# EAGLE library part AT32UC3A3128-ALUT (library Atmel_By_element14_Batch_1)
32-bit Microcontroller
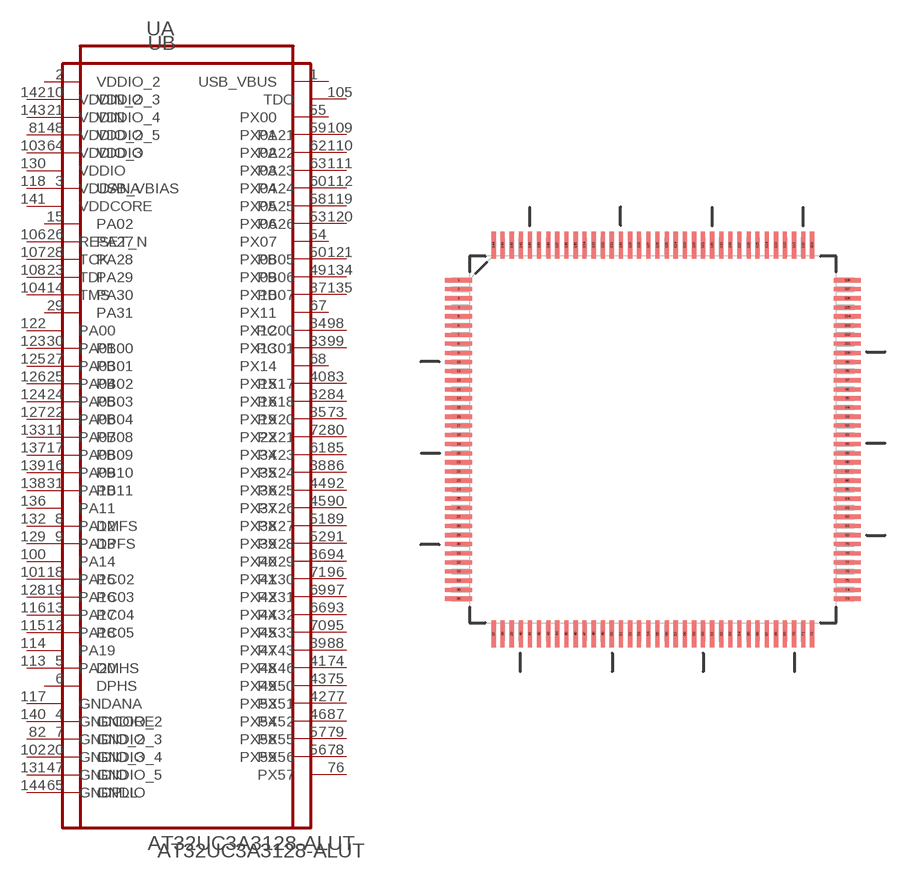
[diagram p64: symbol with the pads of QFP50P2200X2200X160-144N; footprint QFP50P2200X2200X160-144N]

Designator prefix U; gates A=AT32UC3A3128-ALUT_A B=AT32UC3A3128-ALUT_B

## AT32UC3A3128-ALUT (DESCRIPTION: 32-bit Microcontroller; MPN: AT32UC3A3128-ALUT; OC_FARNELL: 1841638; OC_NEWARK: 12T1371; PACKAGE: LQFP-144; SUPPLIER: Atmel Corporation)  [QFP50P2200X2200X160-144N]
1  A:USB_VBUS  out
2  A:VDDIO_2  pwr
3  A:USB_VBIAS  pas
4  A:GNDIO_2  pas
5  A:DMHS  pas
6  A:DPHS  pas
7  A:GNDIO_3  pas
8  A:DMFS
9  A:DPFS
10  A:VDDIO_3  pwr
11  A:PB08
12  A:PC05
13  A:PC04
14  A:PA30
15  A:PA02
16  A:PB10
17  A:PB09
18  A:PC02
19  A:PC03
20  A:GNDIO_4  pas
21  A:VDDIO_4  pwr
22  A:PB04
23  A:PA29
24  A:PB03
25  A:PB02
26  A:PA27
27  A:PB01
28  A:PA28
29  A:PA31
30  A:PB00
31  A:PB11
32  A:PX16
33  A:PX13
34  A:PX12
35  A:PX19
36  A:PX40
37  A:PX10
38  A:PX35
39  A:PX47
40  A:PX15
41  A:PX48
42  A:PX53
43  A:PX49
44  A:PX36
45  A:PX37
46  A:PX54
47  A:GNDIO_5  pas
48  A:VDDIO_5  pwr
49  A:PX09
50  A:PX08
51  A:PX38
52  A:PX39
53  A:PX06
54  A:PX07
55  A:PX00
56  A:PX59
57  A:PX58
58  A:PX05
59  A:PX01
60  A:PX04
61  A:PX34
62  A:PX02
63  A:PX03
64  A:VDDIO  pwr
65  A:GNDIO  pas
66  A:PX44
67  A:PX11
68  A:PX14
69  A:PX42
70  A:PX45
71  A:PX41
72  A:PX22
73  B:PX20
74  B:PX46
75  B:PX50
76  B:PX57
77  B:PX51
78  B:PX56
79  B:PX55
80  B:PX21
81  B:VDDIO_2  pwr
82  B:GNDIO_2  pas
83  B:PX17
84  B:PX18
85  B:PX23
86  B:PX24
87  B:PX52
88  B:PX43
89  B:PX27
90  B:PX26
91  B:PX28
92  B:PX25
93  B:PX32
94  B:PX29
95  B:PX33
96  B:PX30
97  B:PX31
98  B:PC00
99  B:PC01
100  B:PA14
101  B:PA15
102  B:GNDIO_3  pas
103  B:VDDIO_3  pwr
104  B:TMS  in
105  B:TDO  out
106  B:RESET_N  in
107  B:TCK  in
108  B:TDI  in
109  B:PA21
110  B:PA22
111  B:PA23
112  B:PA24
113  B:PA20
114  B:PA19
115  B:PA18
116  B:PA17
117  B:GNDANA  pas
118  B:VDDANA  pwr
119  B:PA25
120  B:PA26
121  B:PB05
122  B:PA00
123  B:PA01
124  B:PA05
125  B:PA03
126  B:PA04
127  B:PA06
128  B:PA16
129  B:PA13
130  B:VDDIO  pwr
131  B:GNDIO  pas
132  B:PA12
133  B:PA07
134  B:PB06
135  B:PB07
136  B:PA11
137  B:PA08
138  B:PA10
139  B:PA09
140  B:GNDCORE  pas
141  B:VDDCORE  pwr
142  B:VDDIN_2  pwr
143  B:VDDIN  pwr
144  B:GNDPLL  pas

## Footprint QFP50P2200X2200X160-144N (pad centres in mm)
smd 1.473 x 0.229: 1 -10.668,8.738; 2 -10.668,8.255; 3 -10.668,7.747; 4 -10.668,7.239; 5 -10.668,6.756; 6 -10.668,6.248; 7 -10.668,5.74; 8 -10.668,5.258; 9 -10.668,4.75; 10 -10.668,4.242; 11 -10.668,3.759; 12 -10.668,3.251; 13 -10.668,2.743; 14 -10.668,2.261; 15 -10.668,1.753; 16 -10.668,1.245; 17 -10.668,0.762; 18 -10.668,0.254; 19 -10.668,-0.254; 20 -10.668,-0.762; 21 -10.668,-1.245; 22 -10.668,-1.753; 23 -10.668,-2.261; 24 -10.668,-2.743; 25 -10.668,-3.251; 26 -10.668,-3.759; 27 -10.668,-4.242; 28 -10.668,-4.75; 29 -10.668,-5.258; 30 -10.668,-5.74; 31 -10.668,-6.248; 32 -10.668,-6.756; 33 -10.668,-7.239; 34 -10.668,-7.747; 35 -10.668,-8.255; 36 -10.668,-8.738; 73 10.668,-8.738; 74 10.668,-8.255; 75 10.668,-7.747; 76 10.668,-7.239; 77 10.668,-6.756; 78 10.668,-6.248; 79 10.668,-5.74; 80 10.668,-5.258; 81 10.668,-4.75; 82 10.668,-4.242; 83 10.668,-3.759; 84 10.668,-3.251; 85 10.668,-2.743; 86 10.668,-2.261; 87 10.668,-1.753; 88 10.668,-1.245; 89 10.668,-0.762; 90 10.668,-0.254; 91 10.668,0.254; 92 10.668,0.762; 93 10.668,1.245; 94 10.668,1.753; 95 10.668,2.261; 96 10.668,2.743; 97 10.668,3.251; 98 10.668,3.759; 99 10.668,4.242; 100 10.668,4.75; 101 10.668,5.258; 102 10.668,5.74; 103 10.668,6.248; 104 10.668,6.756; 105 10.668,7.239; 106 10.668,7.747; 107 10.668,8.255; 108 10.668,8.738
smd 0.229 x 1.473: 37 -8.738,-10.668; 38 -8.255,-10.668; 39 -7.747,-10.668; 40 -7.239,-10.668; 41 -6.756,-10.668; 42 -6.248,-10.668; 43 -5.74,-10.668; 44 -5.258,-10.668; 45 -4.75,-10.668; 46 -4.242,-10.668; 47 -3.759,-10.668; 48 -3.251,-10.668; 49 -2.743,-10.668; 50 -2.261,-10.668; 51 -1.753,-10.668; 52 -1.245,-10.668; 53 -0.762,-10.668; 54 -0.254,-10.668; 55 0.254,-10.668; 56 0.762,-10.668; 57 1.245,-10.668; 58 1.753,-10.668; 59 2.261,-10.668; 60 2.743,-10.668; 61 3.251,-10.668; 62 3.759,-10.668; 63 4.242,-10.668; 64 4.75,-10.668; 65 5.258,-10.668; 66 5.74,-10.668; 67 6.248,-10.668; 68 6.756,-10.668; 69 7.239,-10.668; 70 7.747,-10.668; 71 8.255,-10.668; 72 8.738,-10.668; 109 8.738,10.668; 110 8.255,10.668; 111 7.747,10.668; 112 7.239,10.668; 113 6.756,10.668; 114 6.248,10.668; 115 5.74,10.668; 116 5.258,10.668; 117 4.75,10.668; 118 4.242,10.668; 119 3.759,10.668; 120 3.251,10.668; 121 2.743,10.668; 122 2.261,10.668; 123 1.753,10.668; 124 1.245,10.668; 125 0.762,10.668; 126 0.254,10.668; 127 -0.254,10.668; 128 -0.762,10.668; 129 -1.245,10.668; 130 -1.753,10.668; 131 -2.261,10.668; 132 -2.743,10.668; 133 -3.251,10.668; 134 -3.759,10.668; 135 -4.242,10.668; 136 -4.75,10.668; 137 -5.258,10.668; 138 -5.74,10.668; 139 -6.248,10.668; 140 -6.756,10.668; 141 -7.239,10.668; 142 -7.747,10.668; 143 -8.255,10.668; 144 -8.738,10.668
